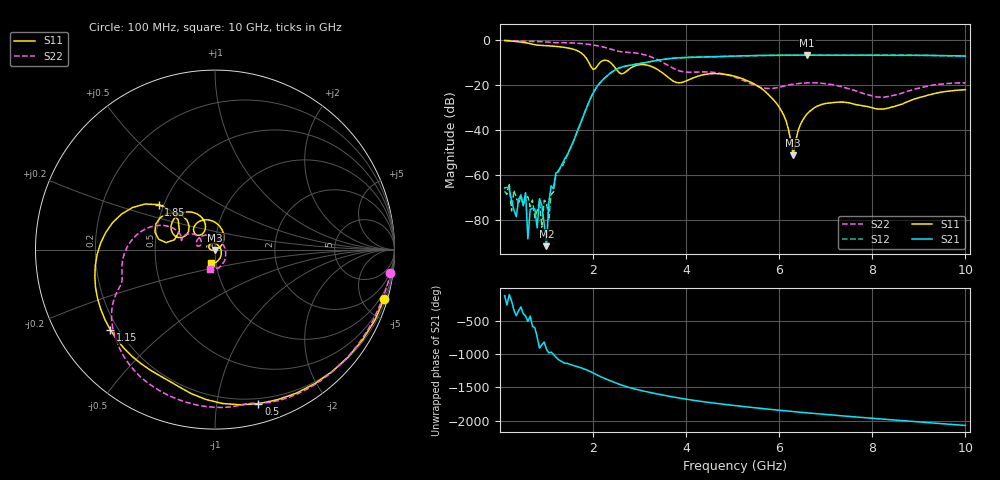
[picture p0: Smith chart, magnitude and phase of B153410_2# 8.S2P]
!  2-Port S-parameters saved by WinCal
! VAR MeasName=S-Parameters (CALIBRATED_DATA) read from VNA (N5245A)
! VAR MeasDate=2016-12-23 9:59:44
! VAR NAME=B153410_2# 8
! VAR FILENAME=B153410_2# 8.S2P
! VAR DATE=2016-12-23 9:59:44
! VAR PHYS_PORTS=1,2
# Hz S DB R 50
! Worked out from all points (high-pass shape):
!   199 points, 100 MHz to 10 GHz, reference 50 ohm
!   highest |S21| = -6.67 dB at 6.6 GHz (marker M1); lowest = -91.8 dB at 1 GHz (marker M2)
!   |S21| within 3 dB of the highest: 3.199 GHz to end of sweep
!   lowest |S11| = -51.4 dB at 6.3 GHz (marker M3), VSWR 1.01, Z = 50.1 - j0.259 ohm
!   |S11| at or under -10 dB: 1.91 GHz to 2.148 GHz (237.2 MHz wide, 11.7 % of centre); 2.375 GHz to end of sweep
!   |S22| runs from -25.4 to -0.1 dB; largest |S21 - S12| = 0.0018
!   S11 on the Smith chart (normalised r, x): 100 MHz: 0.46, -6.99; 500 MHz: 0.16, -1.31; 1.15 GHz: 0.17, -0.33; 1.85 GHz: 0.47, +0.28; 10 GHz: 0.95, -0.14
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1e8  -0.16 -16.2  -65.84 -118.0  -67.35 -132.2  -0.13 -7.4
2.5e8  -0.42 -38.9  -71.70 161.8  -76.16 -134.3  -0.25 -17.6
3.5e8  -0.62 -53.4  -78.66 -61.1  -70.04 114.4  -0.31 -24.3
5e8  -0.99 -74.3  -73.82 -29.8  -73.29 -48.1  -0.39 -34.2
8e8  -2.20 -108.9  -83.64 -23.9  -75.98 -168.4  -0.59 -53.9
8.5e8  -2.30 -113.5  -70.64 171.4  -71.47 133.3  -0.63 -57.2
9e8  -2.36 -118.1  -73.61 -137.7  -83.35 -54.8  -0.68 -60.5
1e9  -2.46 -127.8  -91.79 154.8  -72.30 -146.5  -0.79 -67.1
1.05e9  -2.52 -132.7  -72.30 100.0  -80.04 111.0  -0.87 -70.3
1.15e9  -2.68 -142.6  -66.22 77.6  -67.59 77.5  -1.10 -76.1
1.75e9  -5.76 152.9  -36.15 -127.4  -36.04 -127.0  -1.52 -113.5
1.85e9  -7.92 141.4  -30.65 -153.3  -30.64 -153.3  -1.70 -120.3
2.4e9  -10.43 137.2  -14.26 31.1  -14.25 30.9  -4.12 -154.3
3.4e9  -13.25 115.7  -8.91 -161.7  -8.91 -161.7  -8.86 158.5
4.2e9  -16.44 140.4  -7.59 101.1  -7.59 101.0  -14.23 164.8
5.05e9  -16.14 92.5  -7.10 25.7  -7.11 25.7  -16.49 144.6
5.95e9  -28.34 31.1  -6.74 -41.0  -6.73 -41.0  -21.21 166.0
6.3e9  -51.36 -73.0  -6.69 -64.7  -6.69 -64.5  -19.63 166.9
6.6e9  -32.84 -177.7  -6.67 -83.7  -6.68 -83.7  -19.03 157.1
6.7e9  -31.03 174.7  -6.67 -90.0  -6.68 -90.0  -18.95 153.0
8.35e9  -30.22 12.8  -6.71 175.1  -6.69 175.2  -25.05 7.6
1e10  -22.04 -106.0  -7.09 86.6  -7.09 86.8  -19.04 -104.6
